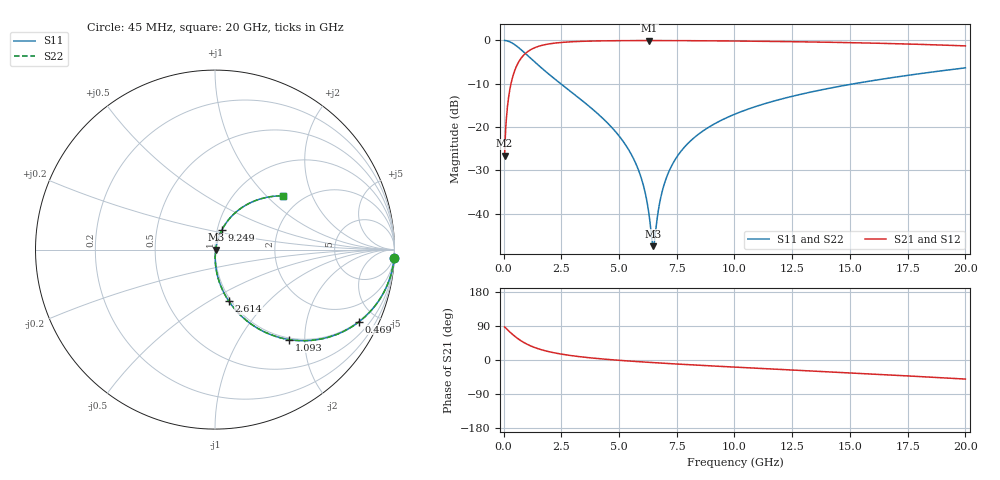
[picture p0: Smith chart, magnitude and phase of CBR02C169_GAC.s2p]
! S-parameter model data by Modelithics Inc.  support@modelithics.com 813-866-6335  Tampa FL USA
! S-Parameter data specifications:
! Substrate: 20-mil Rogers 4350B, substrate thickness, H=0.508mm, Dielectric constant, Er=3.75
! PCB Mounting Pad Footprint: Pad width, PadW=0.32mm , Pad length, PadL=0.37mm , Pad gap, PadG (edge-to-edge)=0.19mm , Reference planes=0.93mm apart
#  GHz  S  MA  R 50
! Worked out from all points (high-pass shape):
!   801 points, 45 MHz to 20 GHz, reference 50 ohm
!   highest |S21| = -0.04 dB at 6.306 GHz (marker M1); lowest = -26.6 dB at 45 MHz (marker M2)
!   |S21| within 3 dB of the highest: 940.8 MHz to end of sweep
!   lowest |S11| = -47.5 dB at 6.48 GHz (marker M3), VSWR 1.01, Z = 50.4 - j0.0766 ohm
!   |S11| at or under -10 dB: 2.477 GHz to 15.17 GHz (12.69 GHz wide, 144 % of centre)
!   |S22| runs from -47.5 to 0.0 dB; largest |S21 - S12| = 0
!   S11 on the Smith chart (normalised r, x): 45 MHz: 1, -42; 469 MHz: 0.97, -4.02; 1.093 GHz: 0.97, -1.69; 2.614 GHz: 0.98, -0.61; 9.249 GHz: 1.05, +0.23; 20 GHz: 1.61, +1.26
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0.045  0.9988 -2.7  0.04667 87.2  0.04667 87.2  0.9988 -2.7
0.24455  0.969 -14.5  0.246 75.4  0.246 75.4  0.969 -14.5
0.469044  0.8981 -26.5  0.4389 63.4  0.4389 63.4  0.8981 -26.5
1.092637  0.6507 -50.4  0.7579 39.4  0.7579 39.4  0.6507 -50.4
1.741175  0.4572 -64.4  0.8873 25.3  0.8873 25.3  0.4572 -64.4
2.614206  0.2959 -75.1  0.9526 14.4  0.9526 14.4  0.2959 -75.1
3.387462  0.2038 -81.0  0.976 8.1  0.976 8.1  0.2038 -81.0
4.63465  0.1026 -87.1  0.9911 0.9  0.9911 0.9  0.1026 -87.1
5.457794  0.05257 -88.6  0.9947 -2.8  0.9947 -2.8  0.05257 -88.6
5.981612  0.02495 -85.7  0.9955 -5.0  0.9955 -5.0  0.02495 -85.7
6.305881  0.009535 -70.3  0.9957 -6.3  0.9957 -6.3  0.009535 -70.3
6.480487  0.004239 -10.3  0.9956 -6.9  0.9956 -6.9  0.004239 -10.3
6.555319  0.005361 30.2  0.9956 -7.2  0.9956 -7.2  0.005361 30.2
6.704981  0.01104 59.2  0.9955 -7.8  0.9955 -7.8  0.01104 59.2
7.004306  0.02402 70.5  0.9952 -8.8  0.9952 -8.8  0.02402 70.5
7.503181  0.04526 73.5  0.9942 -10.6  0.9942 -10.6  0.04526 73.5
8.22655  0.07451 73.2  0.9922 -13.1  0.9922 -13.1  0.07451 73.2
9.249244  0.1134 70.9  0.9881 -16.4  0.9881 -16.4  0.1134 70.9
10.0225  0.1414 68.9  0.9842 -18.8  0.9842 -18.8  0.1414 68.9
13.36496  0.2558 59.3  0.9595 -29.1  0.9595 -29.1  0.2558 59.3
16.68248  0.3674 49.2  0.921 -39.4  0.921 -39.4  0.3674 49.2
20  0.4827 38.4  0.8643 -50.3  0.8643 -50.3  0.4827 38.4
